(* Logix 5000 AddOnInstructionDefinition export Banner_LCA_Param_v4; software revision 33.00 *)

TYPE Banner_IOL_Port_v4 :   // UDT that has all of the data items necessary to communicate with a specific Port on a IO-Link Master
STRUCT
   Port_Controlled : INT;   // Each bit represents a port on an IO-Link Master. Set to 1 to tell AOI to control that port.
   Port_Activate : INT;   // Each bit represents a port on an IO-Link Master. When ON that port will process any commands in queue.
   Port_Read : INT;   // Each bit represents a port on an IO-Link Master. Used to determine when device AOI has requested a Read command.
   Port_Write : INT;   // Each bit represents a port on an IO-Link Master. Used to determine when device AOI has requested a Write command.
   Port_RW_Complete : INT;   // Each bit represents a port on an IO-Link Master. Tells device AOI that Read or Write request has been completed.
   Port_Device_Read : INT;
   Data_Transfer : SINT[190];   // Array to transfer data from IO-Master to device AOIs.
END_STRUCT
END_TYPE

TYPE Banner_LCA_Output_Settings_v4 :
STRUCT
   State : SINT;   // 0 = Normally Closed, 1 = Normally Open
   Off_Delay_Type : SINT;   // 0 = Leading Edge, 1 = Trailing Edge.
   Off_Delay : DINT;   // 0 to 65535 ms.
END_STRUCT
END_TYPE

TYPE Banner_LCA_RD_v4 :   // UDT with all of the Read only parameters for LCA.
STRUCT
   Master_Cycle_Time : INT;
   Min_Cycle_Time : INT;
   M_Sequence_Capability : INT;
   IO_Link_Version_ID : INT;
   Process_Data_Input_Length : INT;
   Process_Data_Output_Length : INT;
   Combined_Vendor_ID : DINT;   // IO-Link Vendor ID
   Vendor_ID1 : INT;
   Vendor_ID2 : INT;
   Combined_Device_ID : DINT;   // IO-Link Device ID
   Device_ID1 : INT;
   Device_ID2 : INT;
   Device_ID3 : INT;
   Serial_Number : STRING;
END_STRUCT
END_TYPE

TYPE Banner_LCA_Settings_v4 :
STRUCT
   Custom_Intensity : SINT;   // 0 to 100 %
   Custom_Flash_Rate : INT;   // Range 5 to 255 (.5 to 25.5 converted rate).
   Restrict_to_Gamut : SINT;   // 0 = Off, 1 = On.
END_STRUCT
END_TYPE

TYPE Banner_LCA_SP_Param_v4 :   // UDT for LCA with the Off State Parameters structure.
STRUCT
   Type : SINT;   // 0 = Off, 1 = Steady, 2 = Flash, 3 = Two Color Flash, 4 = Intensity Sweep, 5 = Color Sweep.
   Output : SINT;   // 0 = Off, 1 = On, 2 = Pattern.
   Pattern : SINT;   // 0 = Flash, 1 = Strobe, 2 = Three Pulse, 3 = SOS, 4 = Random.
   Speed : SINT;   // 0 = Slow, 1 = Medium, 2 = Fast, 3 = Custom.
   Off_Delay_Type : SINT;   // 0 = Leading Edge, 1 = Trailing Edge.
   Off_Delay : DINT;   // 0 to 65535 in ms. Length of time before the device returns to 'touch inactive' state after button is released.
   Color_1 : SINT;   // 0 = Green, 1 = Red, 2 = Orange, 3 = Amber, 4 = Yellow, 5 = Lime Green, 6 = Spring Green, 7 = Cyan, 8 = SKy Blue, 9 = Blue, 10 = Violet, 11 = Magenta, 12 = Rose, 13 = White, 14 Custom 1, 15 = Custom 2.
   Color_1_Intensity : SINT;   // 0 = High, 1 = Medium, 2 = Low, 3 = Off, 4 = Custom.
   Color_2 : SINT;   // 0 = Green, 1 = Red, 2 = Orange, 3 = Amber, 4 = Yellow, 5 = Lime Green, 6 = Spring Green, 7 = Cyan, 8 = SKy Blue, 9 = Blue, 10 = Violet, 11 = Magenta, 12 = Rose, 13 = White, 14 Custom 1, 15 = Custom 2.
   Color_2_Intensity : SINT;   // 0 = High, 1 = Medium, 2 = Low, 3 = Off, 4 = Custom.
END_STRUCT
END_TYPE

TYPE Banner_LCA_SP_v4 :
STRUCT
   Off : Banner_LCA_SP_Param_v4;
   On : Banner_LCA_SP_Param_v4;
   Hold : Banner_LCA_SP_Param_v4;
END_STRUCT
END_TYPE

TYPE Banner_LCA_Touch_Settings_v4 :
STRUCT
   Touch_Sensitivity : SINT;   // 0 = Low, 1 = High.
   Function : SINT[6];   // 0 = Momentary, 1 = Latched.
   Hold : SINT[6];   // 0 = Disabled, 1 = Enabled.
END_STRUCT
END_TYPE

TYPE Banner_LCA_v4 :   // UDT with all of the parameters for LCA.
STRUCT
   Initial_Global_Read : BOOL;   // Determines if all of the IO-Link data has been read into the PLC yet
   Command : INT;   // Value placed in here will activate a read or write to a specifc IO-Link Index
   Read : Banner_LCA_RD_v4;   // All read data
   Write : Banner_LCA_WD_v4;   // All data that can be written to.
   Archive : Banner_LCA_WD_v4;   // Archive of the write data.
   Reset : BOOL;
END_STRUCT
END_TYPE

TYPE Banner_LCA_WD_v4 :   // UDT that stores the Write Data for a LCA.
STRUCT
   System_Command : INT;   // See IODD file for list of commands that can be activated via the System Command interface
   Parameter_Access_Lock : SINT;   // Write access to all read/write parameters is block when this bit is ON.
   Data_Storage_Lock : SINT;   // Data storage mechanism is inhibited when bit is ON.
   Local_Parameterization_Lock : SINT;   // Parameteriation via local control elementes is inhibited.
   Local_User_Interface_Lock : SINT;   // Operation of the hmi on the device is disabled.
   Operation_Mode : SINT;   // 0 = Multicolor, 1 = Four State Full Logic, 2 = Advanced, 3 = LED Control, 4 = Demo.
   Animation_Settings : Banner_LCA_Settings_v4;
   Touch_Settings : Banner_LCA_Touch_Settings_v4;
   Output_Settings : Banner_LCA_Output_Settings_v4;
   State_Parameters : Banner_LCA_SP_v4[6];   // State Parameters. 1 through 5 will have values.
   CC1_Red : INT;   // 0-255. Custom 1 Red.
   CC1_Green : INT;   // 0-255. Custom 1 Green.
   CC1_Blue : INT;   // 0-255. Custom 1 Blue.
   CC2_Red : INT;   // 0-255. Custom 2 Red.
   CC2_Green : INT;   // 0-255. Custom 2 Green.
   CC_Blue : INT;   // 0-255. Custom 2 Blue.
END_STRUCT
END_TYPE

ADD_ON_INSTRUCTION Banner_LCA_Param_SP_In_v4   (* revision 4.0 *)
VAR_INPUT
   Byte1 : SINT; {required}
   Byte2 : SINT; {required}
   Byte3 : SINT; {required}
   Byte4 : SINT; {required}
   Byte5 : SINT; {required}
   Byte6 : SINT; {required}
END_VAR
VAR_IN_OUT
   Data : Banner_LCA_SP_Param_v4; {required}
END_VAR

ROUTINE Logic   (* ladder *)
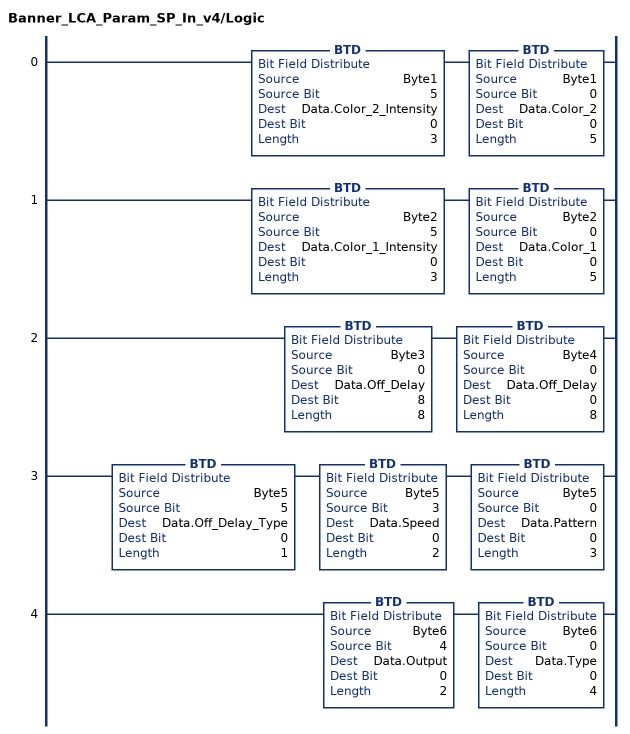
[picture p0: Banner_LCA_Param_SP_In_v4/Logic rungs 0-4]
   0: BTD(Byte1,5,Data.Color_2_Intensity,0,3)BTD(Byte1,0,Data.Color_2,0,5);
   1: BTD(Byte2,5,Data.Color_1_Intensity,0,3)BTD(Byte2,0,Data.Color_1,0,5);
   2: BTD(Byte3,0,Data.Off_Delay,8,8)BTD(Byte4,0,Data.Off_Delay,0,8);
   3: BTD(Byte5,5,Data.Off_Delay_Type,0,1)BTD(Byte5,3,Data.Speed,0,2)BTD(Byte5,0,Data.Pattern,0,3);
   4: BTD(Byte6,4,Data.Output,0,2)BTD(Byte6,0,Data.Type,0,4);
END_ROUTINE
END_ADD_ON_INSTRUCTION

ADD_ON_INSTRUCTION Banner_LCA_Param_SP_Out_v4   (* revision 4.0 *)
VAR_OUTPUT
   Byte1 : SINT; {required}
   Byte2 : SINT; {required}
   Byte3 : SINT; {required}
   Byte4 : SINT; {required}
   Byte5 : SINT; {required}
   Byte6 : SINT; {required}
END_VAR
VAR_IN_OUT
   Data : Banner_LCA_SP_Param_v4; {required}
END_VAR

ROUTINE Logic   (* ladder *)
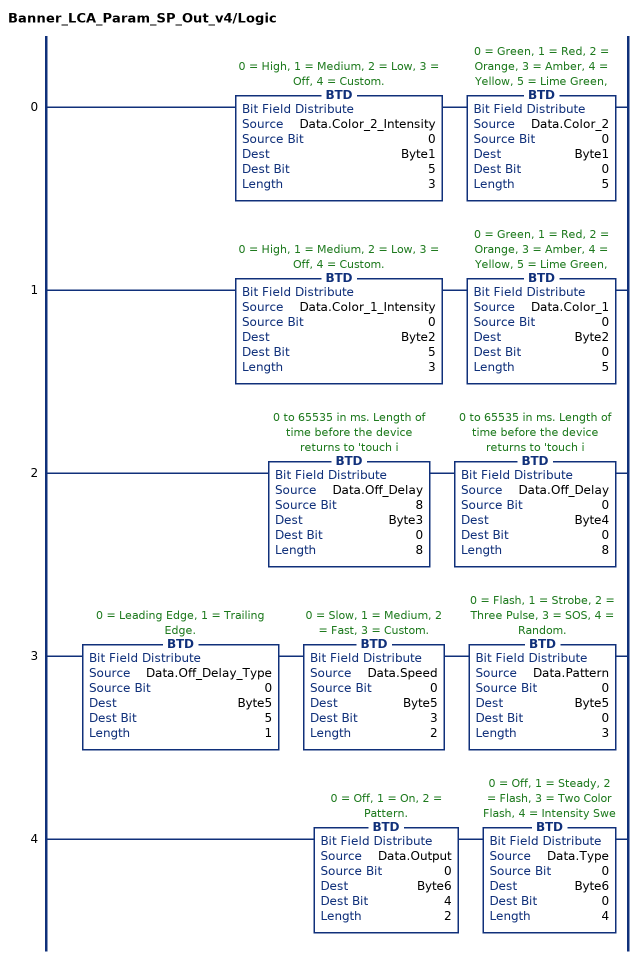
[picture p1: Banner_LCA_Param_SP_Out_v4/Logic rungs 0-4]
   0: BTD(Data.Color_2_Intensity,0,Byte1,5,3)BTD(Data.Color_2,0,Byte1,0,5);
   1: BTD(Data.Color_1_Intensity,0,Byte2,5,3)BTD(Data.Color_1,0,Byte2,0,5);
   2: BTD(Data.Off_Delay,8,Byte3,0,8)BTD(Data.Off_Delay,0,Byte4,0,8);
   3: BTD(Data.Off_Delay_Type,0,Byte5,5,1)BTD(Data.Speed,0,Byte5,3,2)BTD(Data.Pattern,0,Byte5,0,3);
   4: BTD(Data.Output,0,Byte6,4,2)BTD(Data.Type,0,Byte6,0,4);
END_ROUTINE
END_ADD_ON_INSTRUCTION

ADD_ON_INSTRUCTION Banner_LCA_Param_v4   (* revision 4.0, vendor Banner Engineering *)
// AOI to read and write parameter data to an IO-Link LCA.
VAR_IN_OUT
   LCA : Banner_LCA_v4; {required}
   Port_Data : Banner_IOL_Port_v4; {required}
END_VAR
VAR_INPUT
   Port : DINT; {required}
END_VAR
VAR
   Local_Control : DINT; {access None}
   Global_Read_Command_Value : INT; {access None}
   Global_Write_Command_Value : INT; {access None}
   Command_Being_Processed : BOOL; {access None}
   Update_Archive : BOOL; {access None}
   Index_Write_Control : DINT; {access None}
   Index_Write_Inprocess : INT; {access None}
   Temp_Excess_Gain : DINT[2]; {access None}
   Inprocess_Index : DINT; {access None}
   SP_Index : DINT; {access None}   // State Parameters Index
   SP_Write_Index : DINT; {access None}
   SP_R_Index : DINT; {access None}
   SP_W_Index : DINT; {access None}
   StatusIn : Banner_LCA_Param_SP_In_v4[3]; {access None}
   OffArchive : DINT; {access None}
   OffData : DINT; {access None}
   HoldData : DINT; {access None}
   HoldArchive : DINT; {access None}
   OnData : DINT; {access None}
   OnArchive : DINT; {access None}
   StatusOut : Banner_LCA_Param_SP_Out_v4[3]; {access None}
   W_SP_Index : DINT; {access None}
END_VAR

ROUTINE Logic   (* ladder *)
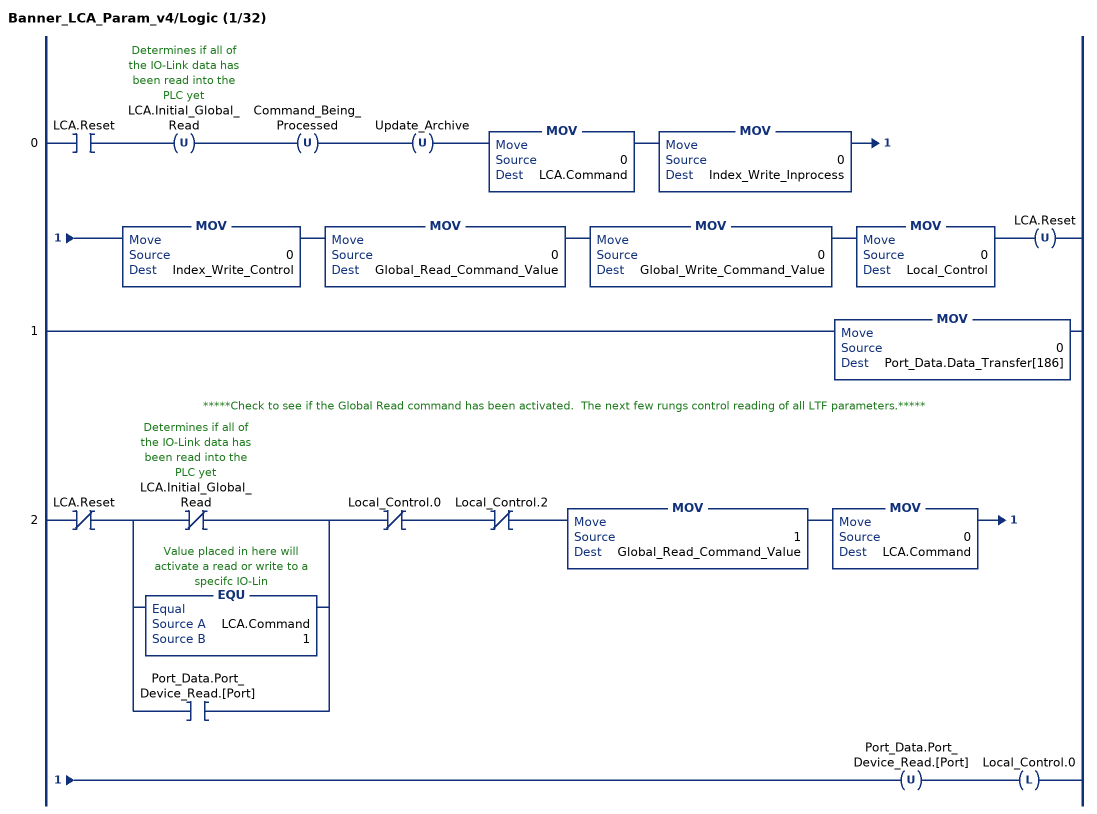
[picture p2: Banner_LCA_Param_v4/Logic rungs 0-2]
   0: XIC(LCA.Reset)OTU(LCA.Initial_Global_Read)OTU(Command_Being_Processed)OTU(Update_Archive)MOV(0,LCA.Command)MOV(0,Index_Write_Inprocess)MOV(0,Index_Write_Control)MOV(0,Global_Read_Command_Value)MOV(0,Global_Write_Command_Value)MOV(0,Local_Control)OTU(LCA.Reset);
   1: MOV(0,Port_Data.Data_Transfer[186]);
   // *****Check to see if the Global Read command has been activated.  The next few rungs control reading of all LTF parameters.*****
   2: XIO(LCA.Reset)[XIO(LCA.Initial_Global_Read) ,EQU(LCA.Command,1) ,XIC(Port_Data.Port_Device_Read.[Port]) ]XIO(Local_Control.0)XIO(Local_Control.2)MOV(1,Global_Read_Command_Value)MOV(0,LCA.Command)OTU(Port_Data.Port_Device_Read.[Port])OTL(Local_Control.0);
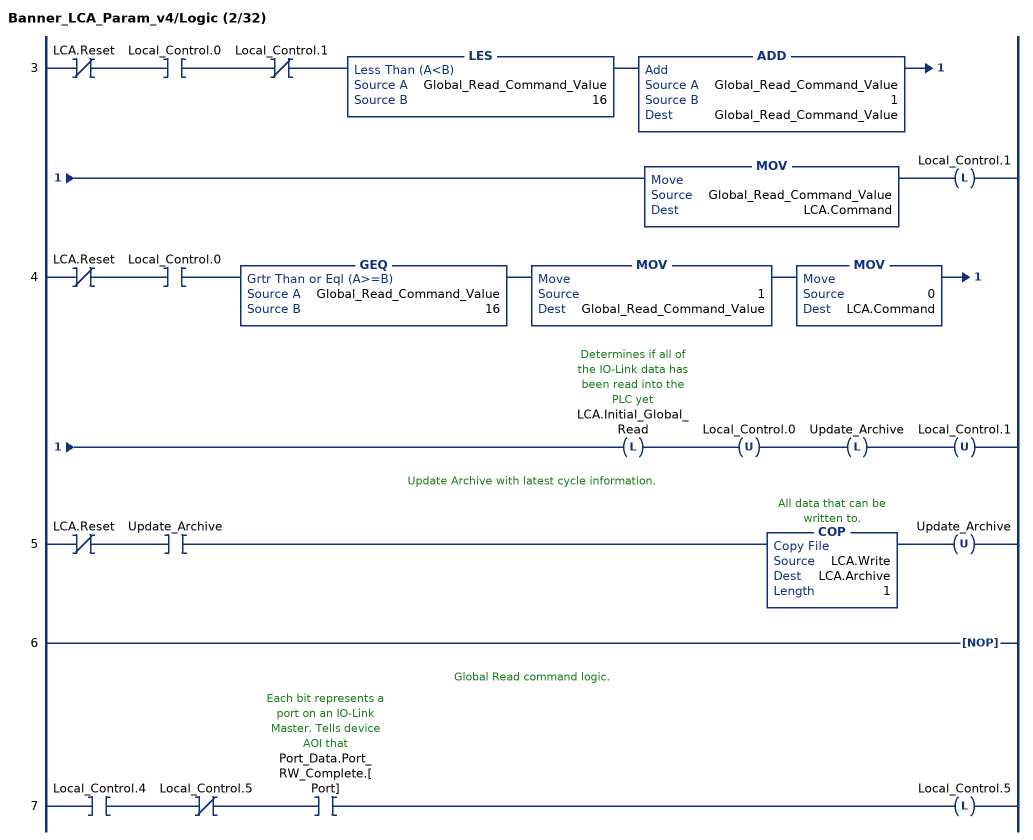
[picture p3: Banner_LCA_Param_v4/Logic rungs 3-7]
   3: XIO(LCA.Reset)XIC(Local_Control.0)XIO(Local_Control.1)LES(Global_Read_Command_Value,16)ADD(Global_Read_Command_Value,1,Global_Read_Command_Value)MOV(Global_Read_Command_Value,LCA.Command)OTL(Local_Control.1);
   4: XIO(LCA.Reset)XIC(Local_Control.0)GEQ(Global_Read_Command_Value,16)MOV(1,Global_Read_Command_Value)MOV(0,LCA.Command)OTL(LCA.Initial_Global_Read)OTU(Local_Control.0)OTL(Update_Archive)OTU(Local_Control.1);
   // Update Archive with latest cycle information.
   5: XIO(LCA.Reset)XIC(Update_Archive)COP(LCA.Write,LCA.Archive,1)OTU(Update_Archive);
   6: NOP();
   // Global Read command logic.
   7: XIC(Local_Control.4)XIO(Local_Control.5)XIC(Port_Data.Port_RW_Complete.[Port])OTL(Local_Control.5);
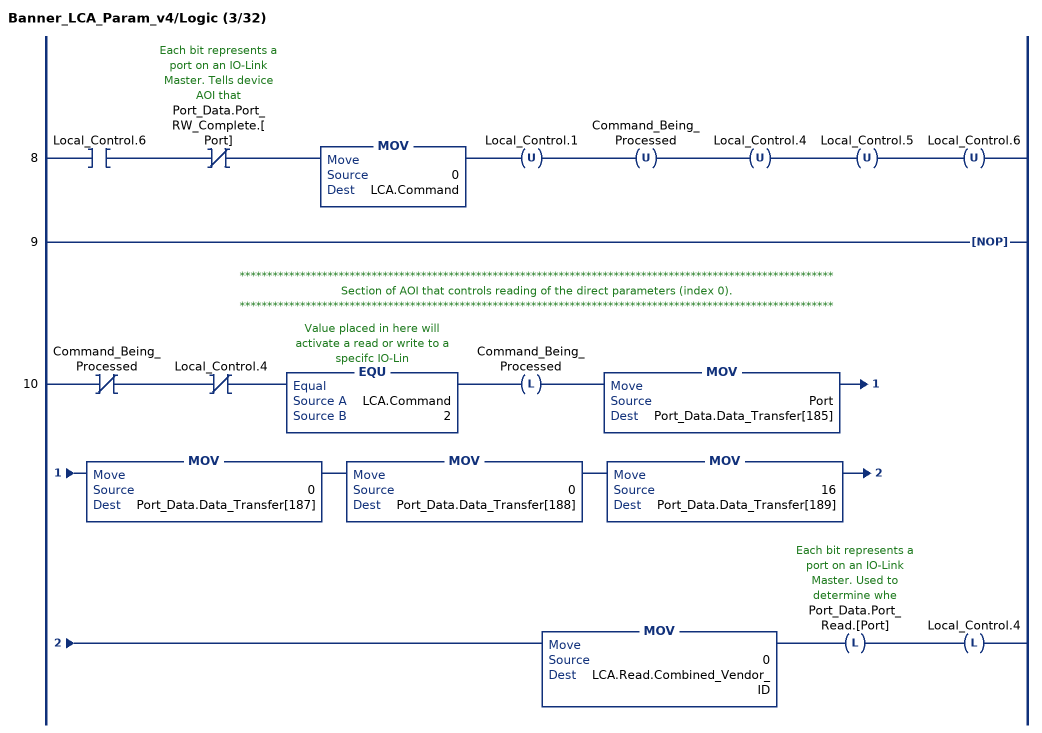
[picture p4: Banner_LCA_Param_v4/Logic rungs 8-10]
   8: XIC(Local_Control.6)XIO(Port_Data.Port_RW_Complete.[Port])MOV(0,LCA.Command)OTU(Local_Control.1)OTU(Command_Being_Processed)OTU(Local_Control.4)OTU(Local_Control.5)OTU(Local_Control.6);
   9: NOP();
   // ************************************************************************************************************
   // Section of AOI that controls reading of the direct parameters (index 0).
   // ************************************************************************************************************
   10: XIO(Command_Being_Processed)XIO(Local_Control.4)EQU(LCA.Command,2)OTL(Command_Being_Processed)MOV(Port,Port_Data.Data_Transfer[185])MOV(0,Port_Data.Data_Transfer[187])MOV(0,Port_Data.Data_Transfer[188])MOV(16,Port_Data.Data_Transfer[189])MOV(0,LCA.Read.Combined_Vendor_ID)OTL(Port_Data.Port_Read.[Port])OTL(Local_Control.4);
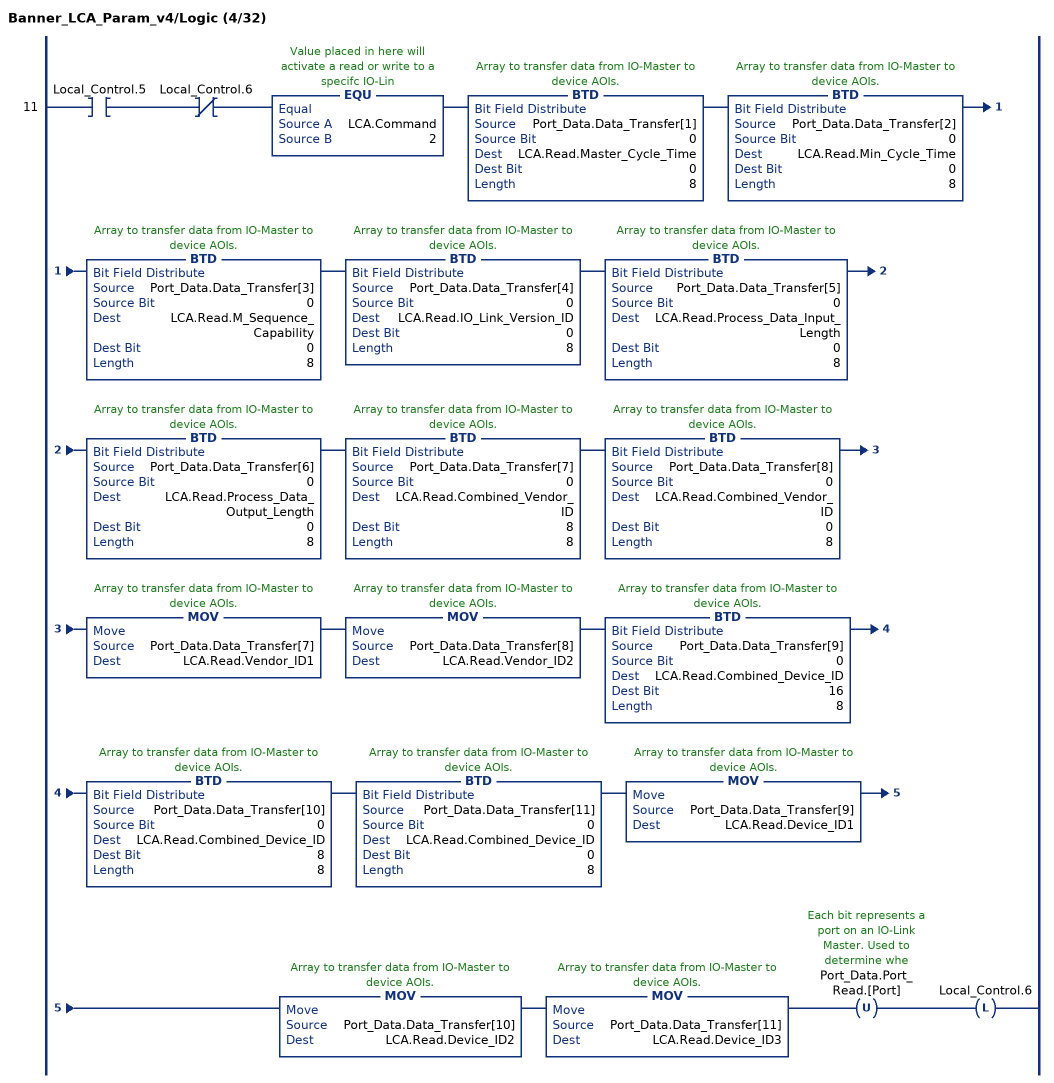
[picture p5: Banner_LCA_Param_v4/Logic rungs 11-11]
   11: XIC(Local_Control.5)XIO(Local_Control.6)EQU(LCA.Command,2)BTD(Port_Data.Data_Transfer[1],0,LCA.Read.Master_Cycle_Time,0,8)BTD(Port_Data.Data_Transfer[2],0,LCA.Read.Min_Cycle_Time,0,8)BTD(Port_Data.Data_Transfer[3],0,LCA.Read.M_Sequence_Capability,0,8)BTD(Port_Data.Data_Transfer[4],0,LCA.Read.IO_Link_Version_ID,0,8)BTD(Port_Data.Data_Transfer[5],0,LCA.Read.Process_Data_Input_Length,0,8)BTD(Port_Data.Data_Transfer[6],0,LCA.Read.Process_Data_Output_Length,0,8)BTD(Port_Data.Data_Transfer[7],0,LCA.Read.Combined_Vendor_ID,8,8)BTD(Port_Data.Data_Transfer[8],0,LCA.Read.Combined_Vendor_ID,0,8)MOV(Port_Data.Data_Transfer[7],LCA.Read.Vendor_ID1)MOV(Port_Data.Data_Transfer[8],LCA.Read.Vendor_ID2)BTD(Port_Data.Data_Transfer[9],0,LCA.Read.Combined_Device_ID,16,8)BTD(Port_Data.Data_Transfer[10],0,LCA.Read.Combined_Device_ID,8,8)BTD(Port_Data.Data_Transfer[11],0,LCA.Read.Combined_Device_ID,0,8)MOV(Port_Data.Data_Transfer[9],LCA.Read.Device_ID1)MOV(Port_Data.Data_Transfer[10],LCA.Read.Device_ID2)MOV(Port_Data.Data_Transfer[11],LCA.Read.Device_ID3)OTU(Port_Data.Port_Read.[Port])OTL(Local_Control.6);
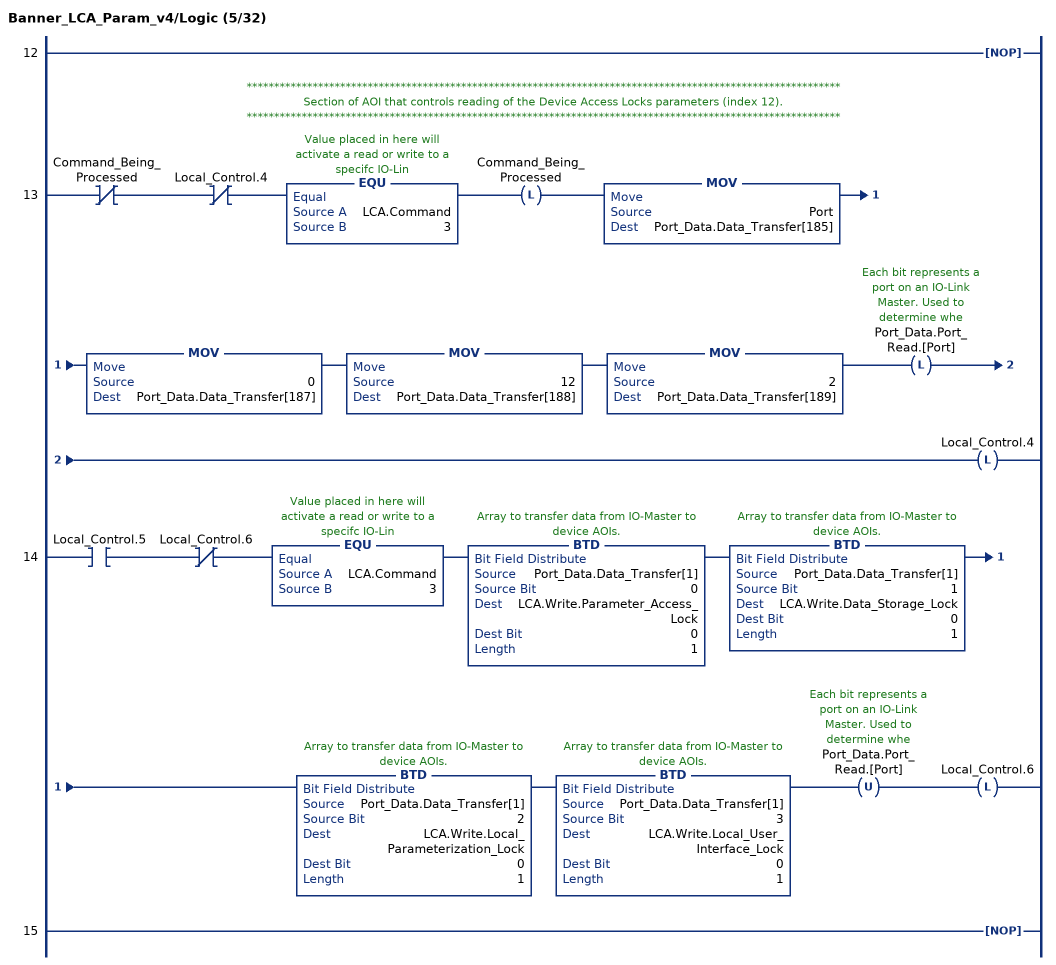
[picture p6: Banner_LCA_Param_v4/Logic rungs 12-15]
   12: NOP();
   // ************************************************************************************************************
   // Section of AOI that controls reading of the Device Access Locks parameters (index 12).
   // ************************************************************************************************************
   13: XIO(Command_Being_Processed)XIO(Local_Control.4)EQU(LCA.Command,3)OTL(Command_Being_Processed)MOV(Port,Port_Data.Data_Transfer[185])MOV(0,Port_Data.Data_Transfer[187])MOV(12,Port_Data.Data_Transfer[188])MOV(2,Port_Data.Data_Transfer[189])OTL(Port_Data.Port_Read.[Port])OTL(Local_Control.4);
   14: XIC(Local_Control.5)XIO(Local_Control.6)EQU(LCA.Command,3)BTD(Port_Data.Data_Transfer[1],0,LCA.Write.Parameter_Access_Lock,0,1)BTD(Port_Data.Data_Transfer[1],1,LCA.Write.Data_Storage_Lock,0,1)BTD(Port_Data.Data_Transfer[1],2,LCA.Write.Local_Parameterization_Lock,0,1)BTD(Port_Data.Data_Transfer[1],3,LCA.Write.Local_User_Interface_Lock,0,1)OTU(Port_Data.Port_Read.[Port])OTL(Local_Control.6);
   15: NOP();
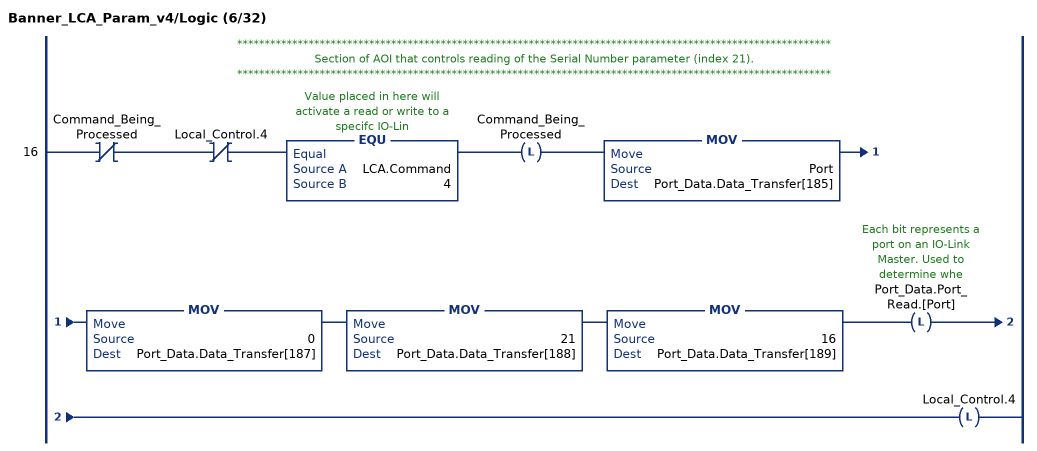
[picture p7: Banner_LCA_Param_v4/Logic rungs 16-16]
   // ************************************************************************************************************
   // Section of AOI that controls reading of the Serial Number parameter (index 21).
   // ************************************************************************************************************
   16: XIO(Command_Being_Processed)XIO(Local_Control.4)EQU(LCA.Command,4)OTL(Command_Being_Processed)MOV(Port,Port_Data.Data_Transfer[185])MOV(0,Port_Data.Data_Transfer[187])MOV(21,Port_Data.Data_Transfer[188])MOV(16,Port_Data.Data_Transfer[189])OTL(Port_Data.Port_Read.[Port])OTL(Local_Control.4);
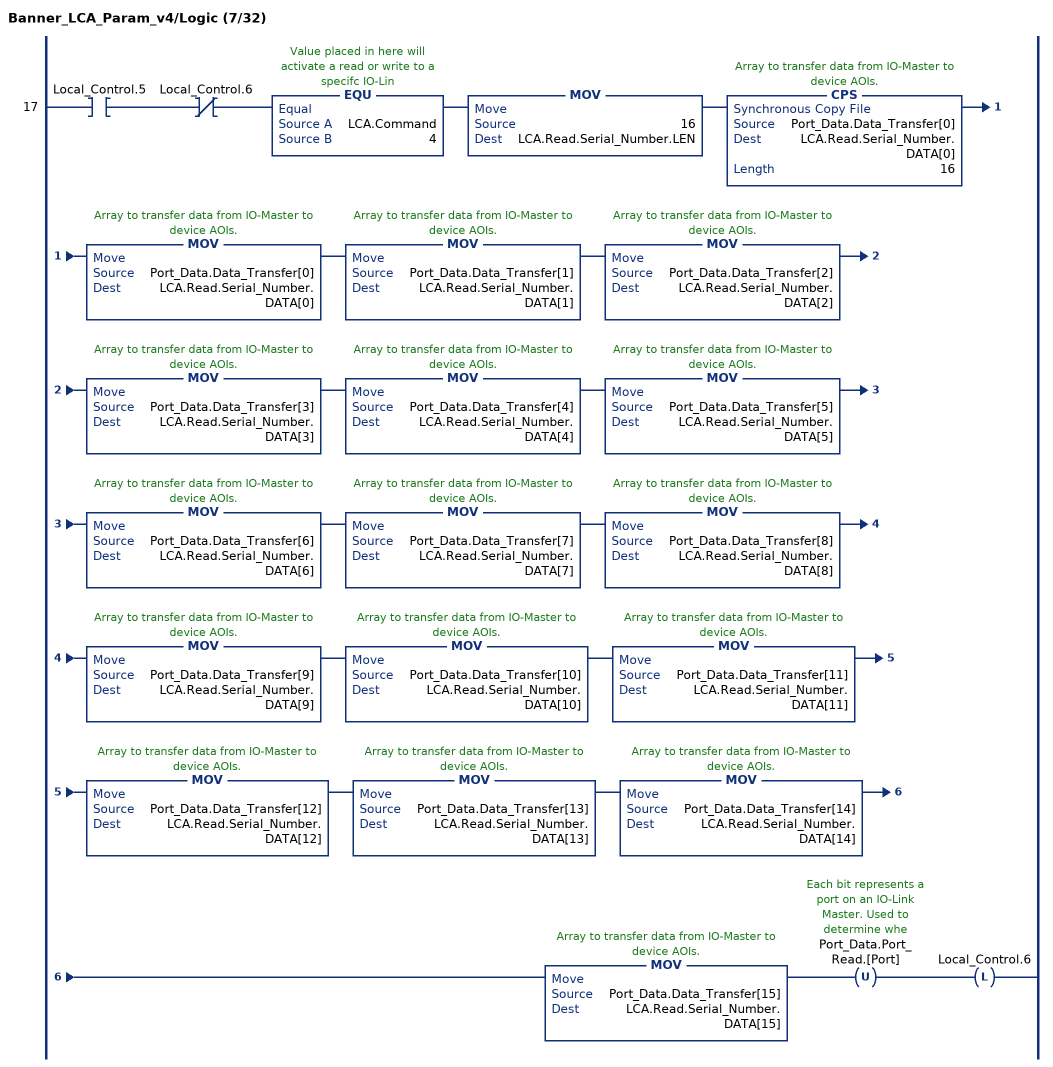
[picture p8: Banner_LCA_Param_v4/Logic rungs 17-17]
   17: XIC(Local_Control.5)XIO(Local_Control.6)EQU(LCA.Command,4)MOV(16,LCA.Read.Serial_Number.LEN)CPS(Port_Data.Data_Transfer[0],LCA.Read.Serial_Number.DATA[0],16)MOV(Port_Data.Data_Transfer[0],LCA.Read.Serial_Number.DATA[0])MOV(Port_Data.Data_Transfer[1],LCA.Read.Serial_Number.DATA[1])MOV(Port_Data.Data_Transfer[2],LCA.Read.Serial_Number.DATA[2])MOV(Port_Data.Data_Transfer[3],LCA.Read.Serial_Number.DATA[3])MOV(Port_Data.Data_Transfer[4],LCA.Read.Serial_Number.DATA[4])MOV(Port_Data.Data_Transfer[5],LCA.Read.Serial_Number.DATA[5])MOV(Port_Data.Data_Transfer[6],LCA.Read.Serial_Number.DATA[6])MOV(Port_Data.Data_Transfer[7],LCA.Read.Serial_Number.DATA[7])MOV(Port_Data.Data_Transfer[8],LCA.Read.Serial_Number.DATA[8])MOV(Port_Data.Data_Transfer[9],LCA.Read.Serial_Number.DATA[9])MOV(Port_Data.Data_Transfer[10],LCA.Read.Serial_Number.DATA[10])MOV(Port_Data.Data_Transfer[11],LCA.Read.Serial_Number.DATA[11])MOV(Port_Data.Data_Transfer[12],LCA.Read.Serial_Number.DATA[12])MOV(Port_Data.Data_Transfer[13],LCA.Read.Serial_Number.DATA[13])MOV(Port_Data.Data_Transfer[14],LCA.Read.Serial_Number.DATA[14])MOV(Port_Data.Data_Transfer[15],LCA.Read.Serial_Number.DATA[15])OTU(Port_Data.Port_Read.[Port])OTL(Local_Control.6);
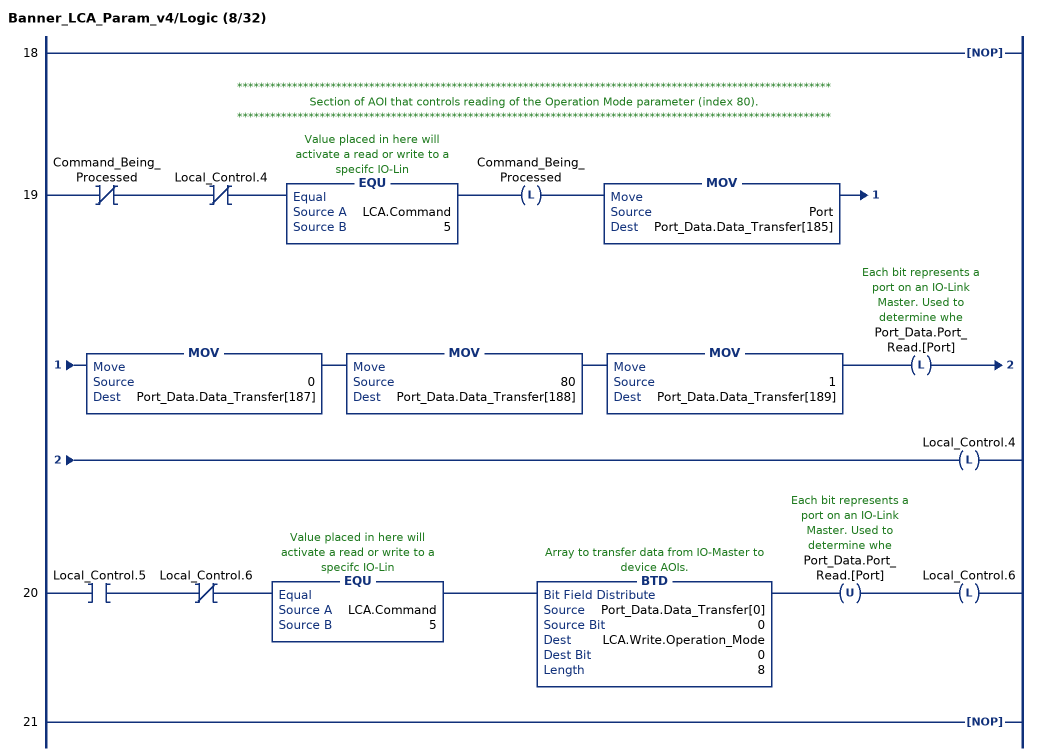
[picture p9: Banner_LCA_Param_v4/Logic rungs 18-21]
   18: NOP();
   // ************************************************************************************************************
   // Section of AOI that controls reading of the Operation Mode parameter (index 80).
   // ************************************************************************************************************
   19: XIO(Command_Being_Processed)XIO(Local_Control.4)EQU(LCA.Command,5)OTL(Command_Being_Processed)MOV(Port,Port_Data.Data_Transfer[185])MOV(0,Port_Data.Data_Transfer[187])MOV(80,Port_Data.Data_Transfer[188])MOV(1,Port_Data.Data_Transfer[189])OTL(Port_Data.Port_Read.[Port])OTL(Local_Control.4);
   20: XIC(Local_Control.5)XIO(Local_Control.6)EQU(LCA.Command,5)BTD(Port_Data.Data_Transfer[0],0,LCA.Write.Operation_Mode,0,8)OTU(Port_Data.Port_Read.[Port])OTL(Local_Control.6);
   21: NOP();
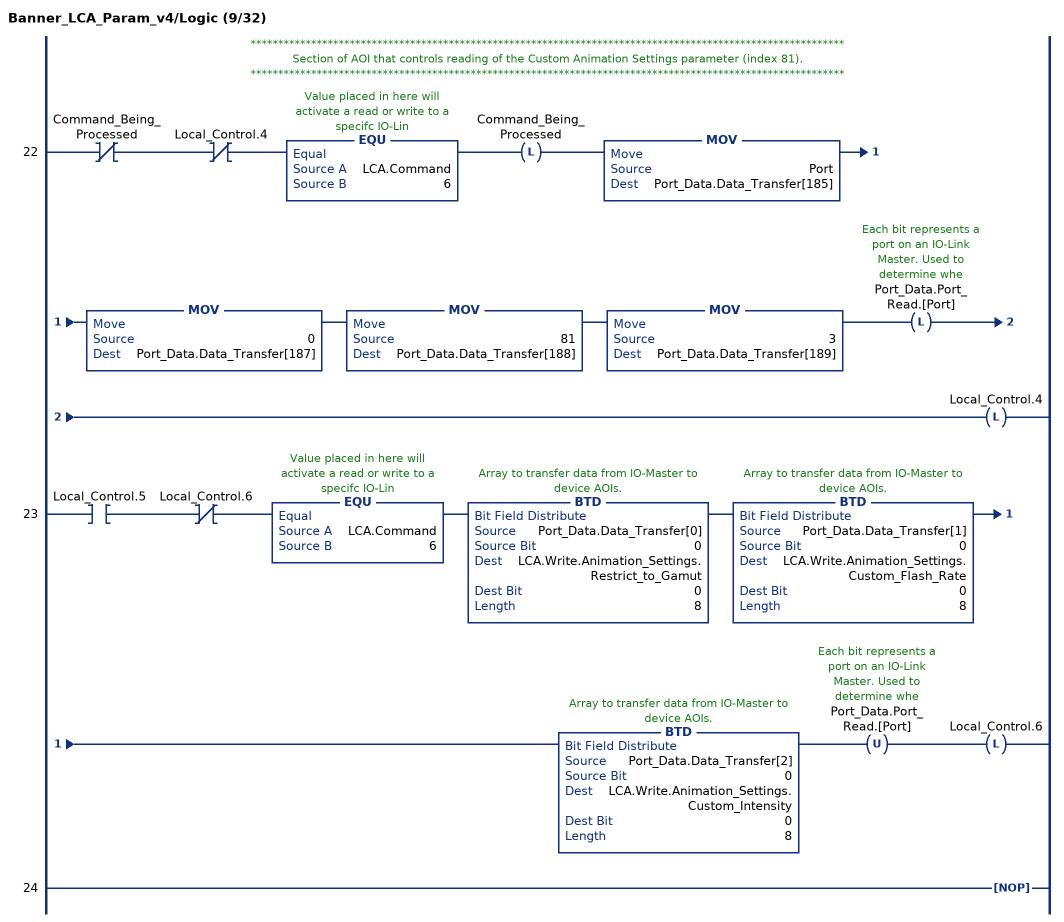
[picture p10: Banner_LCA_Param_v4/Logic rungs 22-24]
   // ************************************************************************************************************
   // Section of AOI that controls reading of the Custom Animation Settings parameter (index 81).
   // ************************************************************************************************************
   22: XIO(Command_Being_Processed)XIO(Local_Control.4)EQU(LCA.Command,6)OTL(Command_Being_Processed)MOV(Port,Port_Data.Data_Transfer[185])MOV(0,Port_Data.Data_Transfer[187])MOV(81,Port_Data.Data_Transfer[188])MOV(3,Port_Data.Data_Transfer[189])OTL(Port_Data.Port_Read.[Port])OTL(Local_Control.4);
   23: XIC(Local_Control.5)XIO(Local_Control.6)EQU(LCA.Command,6)BTD(Port_Data.Data_Transfer[0],0,LCA.Write.Animation_Settings.Restrict_to_Gamut,0,8)BTD(Port_Data.Data_Transfer[1],0,LCA.Write.Animation_Settings.Custom_Flash_Rate,0,8)BTD(Port_Data.Data_Transfer[2],0,LCA.Write.Animation_Settings.Custom_Intensity,0,8)OTU(Port_Data.Port_Read.[Port])OTL(Local_Control.6);
   24: NOP();
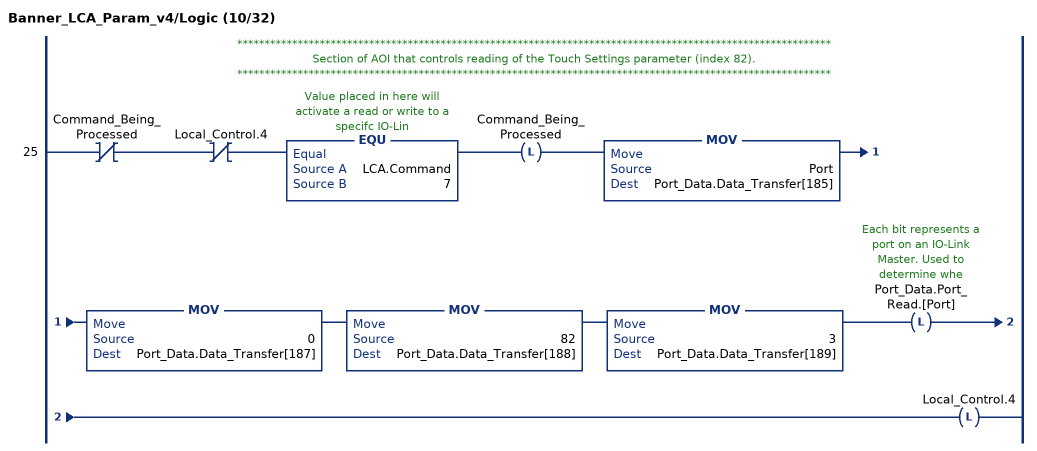
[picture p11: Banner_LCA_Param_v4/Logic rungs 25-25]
   // ************************************************************************************************************
   // Section of AOI that controls reading of the Touch Settings parameter (index 82).
   // ************************************************************************************************************
   25: XIO(Command_Being_Processed)XIO(Local_Control.4)EQU(LCA.Command,7)OTL(Command_Being_Processed)MOV(Port,Port_Data.Data_Transfer[185])MOV(0,Port_Data.Data_Transfer[187])MOV(82,Port_Data.Data_Transfer[188])MOV(3,Port_Data.Data_Transfer[189])OTL(Port_Data.Port_Read.[Port])OTL(Local_Control.4);
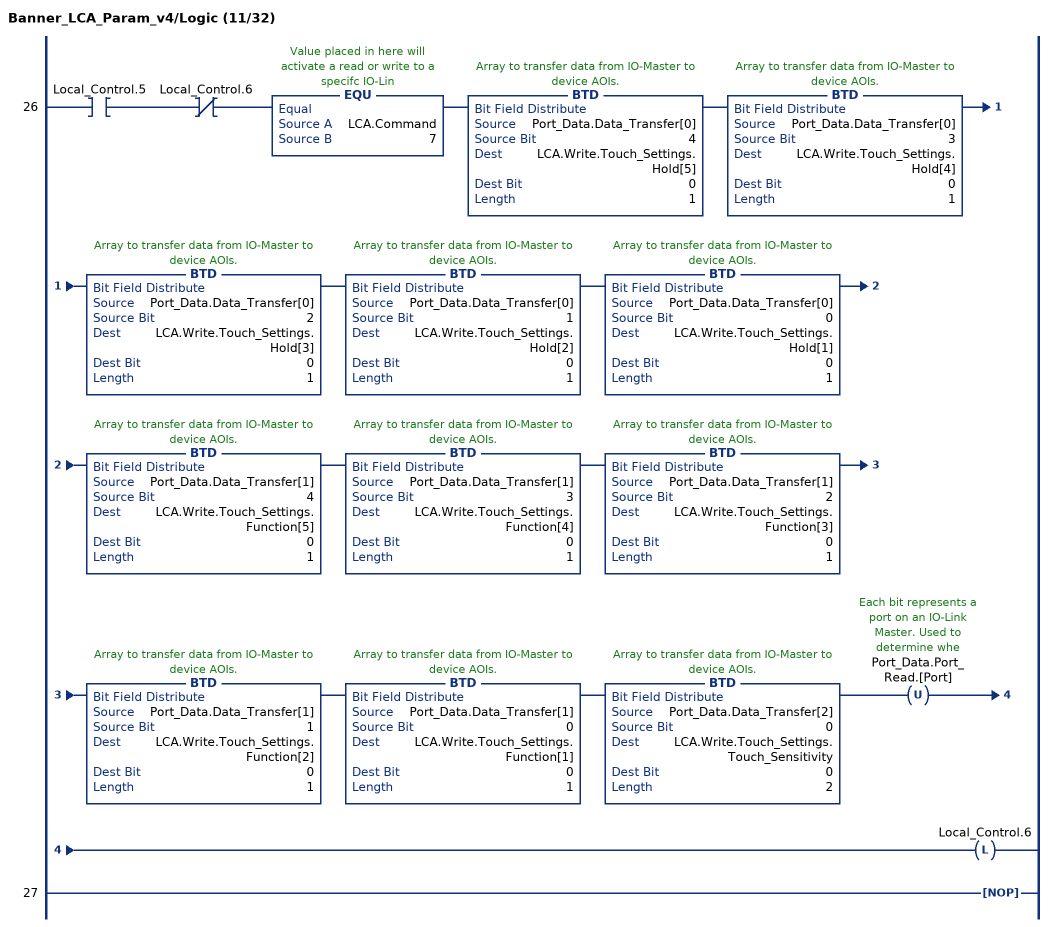
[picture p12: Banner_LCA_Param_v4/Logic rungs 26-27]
   26: XIC(Local_Control.5)XIO(Local_Control.6)EQU(LCA.Command,7)BTD(Port_Data.Data_Transfer[0],4,LCA.Write.Touch_Settings.Hold[5],0,1)BTD(Port_Data.Data_Transfer[0],3,LCA.Write.Touch_Settings.Hold[4],0,1)BTD(Port_Data.Data_Transfer[0],2,LCA.Write.Touch_Settings.Hold[3],0,1)BTD(Port_Data.Data_Transfer[0],1,LCA.Write.Touch_Settings.Hold[2],0,1)BTD(Port_Data.Data_Transfer[0],0,LCA.Write.Touch_Settings.Hold[1],0,1)BTD(Port_Data.Data_Transfer[1],4,LCA.Write.Touch_Settings.Function[5],0,1)BTD(Port_Data.Data_Transfer[1],3,LCA.Write.Touch_Settings.Function[4],0,1)BTD(Port_Data.Data_Transfer[1],2,LCA.Write.Touch_Settings.Function[3],0,1)BTD(Port_Data.Data_Transfer[1],1,LCA.Write.Touch_Settings.Function[2],0,1)BTD(Port_Data.Data_Transfer[1],0,LCA.Write.Touch_Settings.Function[1],0,1)BTD(Port_Data.Data_Transfer[2],0,LCA.Write.Touch_Settings.Touch_Sensitivity,0,2)OTU(Port_Data.Port_Read.[Port])OTL(Local_Control.6);
   27: NOP();
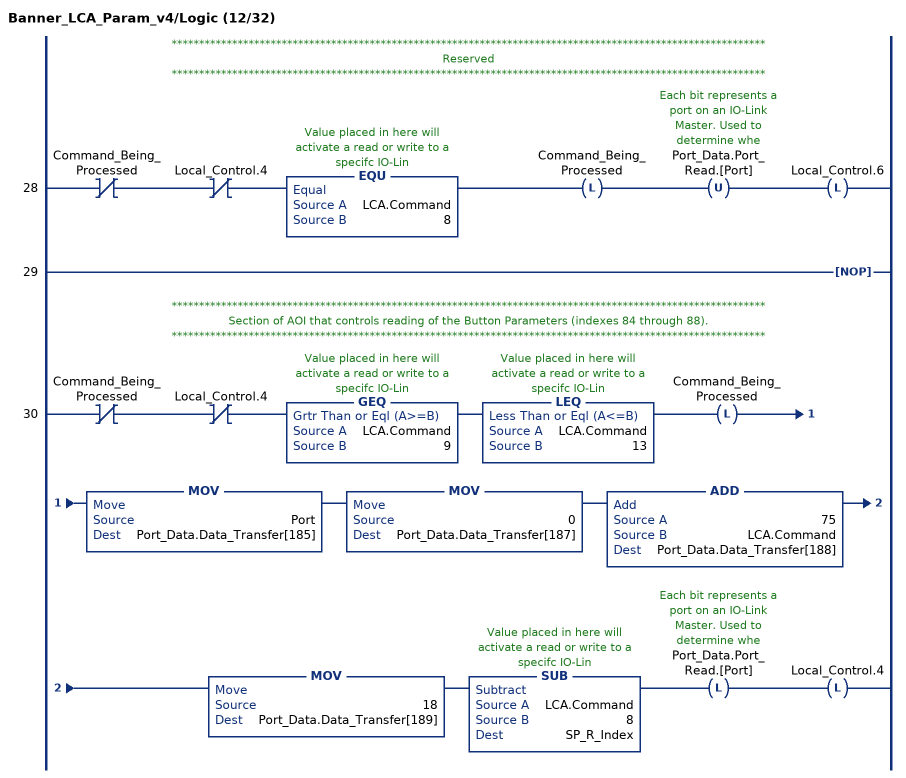
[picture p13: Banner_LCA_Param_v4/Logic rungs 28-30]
   // ************************************************************************************************************
   // Reserved
   // ************************************************************************************************************
   28: XIO(Command_Being_Processed)XIO(Local_Control.4)EQU(LCA.Command,8)OTL(Command_Being_Processed)OTU(Port_Data.Port_Read.[Port])OTL(Local_Control.6);
   29: NOP();
   // ************************************************************************************************************
   // Section of AOI that controls reading of the Button Parameters (indexes 84 through 88).
   // ************************************************************************************************************
   30: XIO(Command_Being_Processed)XIO(Local_Control.4)GEQ(LCA.Command,9)LEQ(LCA.Command,13)OTL(Command_Being_Processed)MOV(Port,Port_Data.Data_Transfer[185])MOV(0,Port_Data.Data_Transfer[187])ADD(75,LCA.Command,Port_Data.Data_Transfer[188])MOV(18,Port_Data.Data_Transfer[189])SUB(LCA.Command,8,SP_R_Index)OTL(Port_Data.Port_Read.[Port])OTL(Local_Control.4);
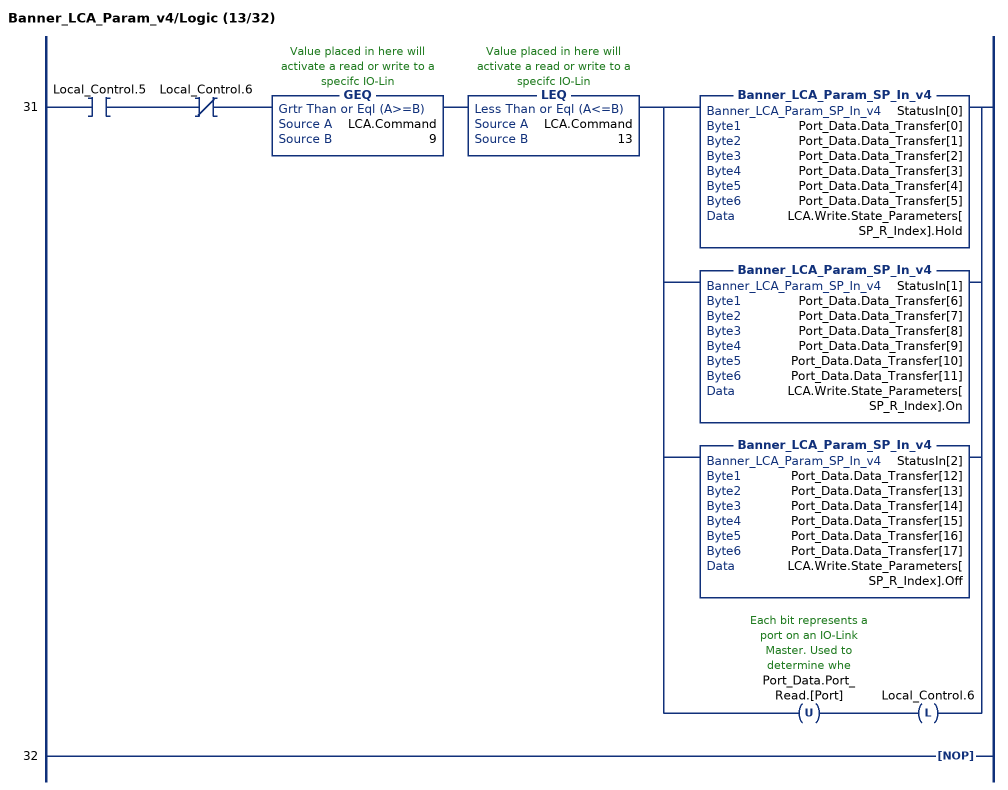
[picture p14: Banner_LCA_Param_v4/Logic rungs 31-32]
   31: XIC(Local_Control.5)XIO(Local_Control.6)GEQ(LCA.Command,9)LEQ(LCA.Command,13)[Banner_LCA_Param_SP_In_v4(StatusIn[0],Port_Data.Data_Transfer[0],Port_Data.Data_Transfer[1],Port_Data.Data_Transfer[2],Port_Data.Data_Transfer[3],Port_Data.Data_Transfer[4],Port_Data.Data_Transfer[5],LCA.Write.State_Parameters[SP_R_Index].Hold) ,Banner_LCA_Param_SP_In_v4(StatusIn[1],Port_Data.Data_Transfer[6],Port_Data.Data_Transfer[7],Port_Data.Data_Transfer[8],Port_Data.Data_Transfer[9],Port_Data.Data_Transfer[10],Port_Data.Data_Transfer[11],LCA.Write.State_Parameters[SP_R_Index].On) ,Banner_LCA_Param_SP_In_v4(StatusIn[2],Port_Data.Data_Transfer[12],Port_Data.Data_Transfer[13],Port_Data.Data_Transfer[14],Port_Data.Data_Transfer[15],Port_Data.Data_Transfer[16],Port_Data.Data_Transfer[17],LCA.Write.State_Parameters[SP_R_Index].Off) ,OTU(Port_Data.Port_Read.[Port]) OTL(Local_Control.6) ];
   32: NOP();
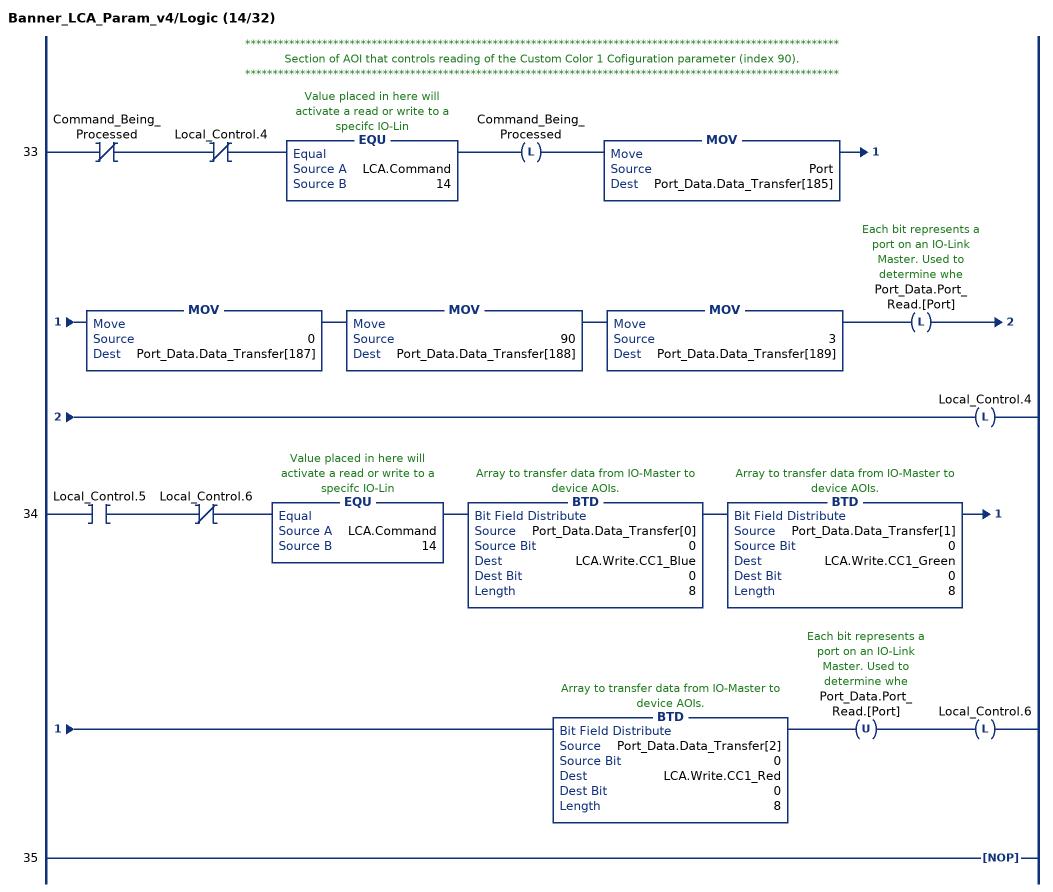
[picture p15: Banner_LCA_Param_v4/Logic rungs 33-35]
   // ************************************************************************************************************
   // Section of AOI that controls reading of the Custom Color 1 Cofiguration parameter (index 90).
   // ************************************************************************************************************
   33: XIO(Command_Being_Processed)XIO(Local_Control.4)EQU(LCA.Command,14)OTL(Command_Being_Processed)MOV(Port,Port_Data.Data_Transfer[185])MOV(0,Port_Data.Data_Transfer[187])MOV(90,Port_Data.Data_Transfer[188])MOV(3,Port_Data.Data_Transfer[189])OTL(Port_Data.Port_Read.[Port])OTL(Local_Control.4);
   34: XIC(Local_Control.5)XIO(Local_Control.6)EQU(LCA.Command,14)BTD(Port_Data.Data_Transfer[0],0,LCA.Write.CC1_Blue,0,8)BTD(Port_Data.Data_Transfer[1],0,LCA.Write.CC1_Green,0,8)BTD(Port_Data.Data_Transfer[2],0,LCA.Write.CC1_Red,0,8)OTU(Port_Data.Port_Read.[Port])OTL(Local_Control.6);
   35: NOP();
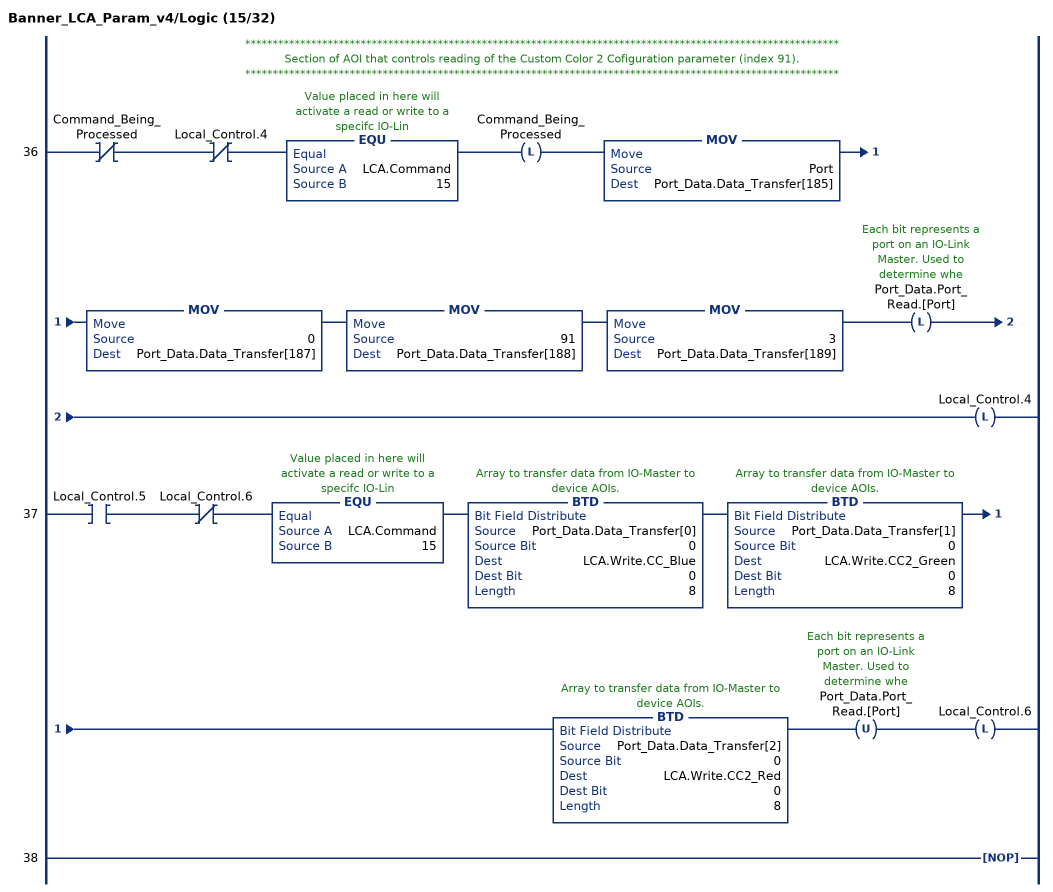
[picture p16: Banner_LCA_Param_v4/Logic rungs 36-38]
   // ************************************************************************************************************
   // Section of AOI that controls reading of the Custom Color 2 Cofiguration parameter (index 91).
   // ************************************************************************************************************
   36: XIO(Command_Being_Processed)XIO(Local_Control.4)EQU(LCA.Command,15)OTL(Command_Being_Processed)MOV(Port,Port_Data.Data_Transfer[185])MOV(0,Port_Data.Data_Transfer[187])MOV(91,Port_Data.Data_Transfer[188])MOV(3,Port_Data.Data_Transfer[189])OTL(Port_Data.Port_Read.[Port])OTL(Local_Control.4);
   37: XIC(Local_Control.5)XIO(Local_Control.6)EQU(LCA.Command,15)BTD(Port_Data.Data_Transfer[0],0,LCA.Write.CC_Blue,0,8)BTD(Port_Data.Data_Transfer[1],0,LCA.Write.CC2_Green,0,8)BTD(Port_Data.Data_Transfer[2],0,LCA.Write.CC2_Red,0,8)OTU(Port_Data.Port_Read.[Port])OTL(Local_Control.6);
   38: NOP();
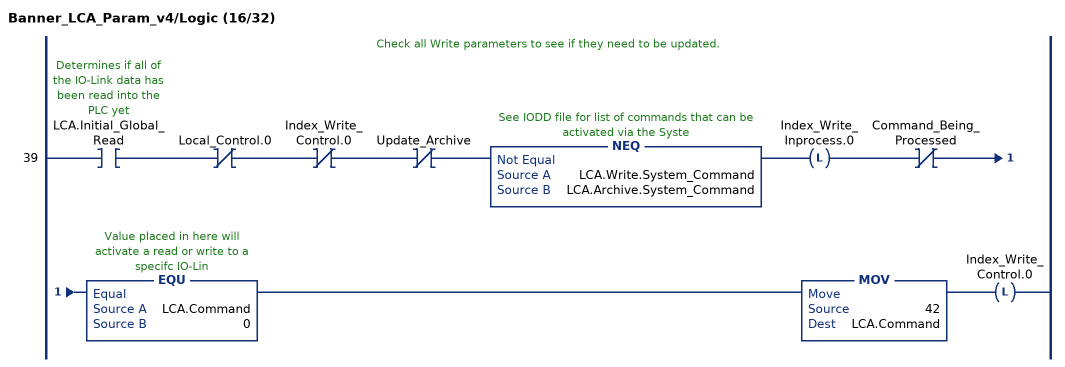
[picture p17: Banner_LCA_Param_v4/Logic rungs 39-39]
   // Check all Write parameters to see if they need to be updated.
   39: XIC(LCA.Initial_Global_Read)XIO(Local_Control.0)XIO(Index_Write_Control.0)XIO(Update_Archive)NEQ(LCA.Write.System_Command,LCA.Archive.System_Command)OTL(Index_Write_Inprocess.0)XIO(Command_Being_Processed)EQU(LCA.Command,0)MOV(42,LCA.Command)OTL(Index_Write_Control.0);
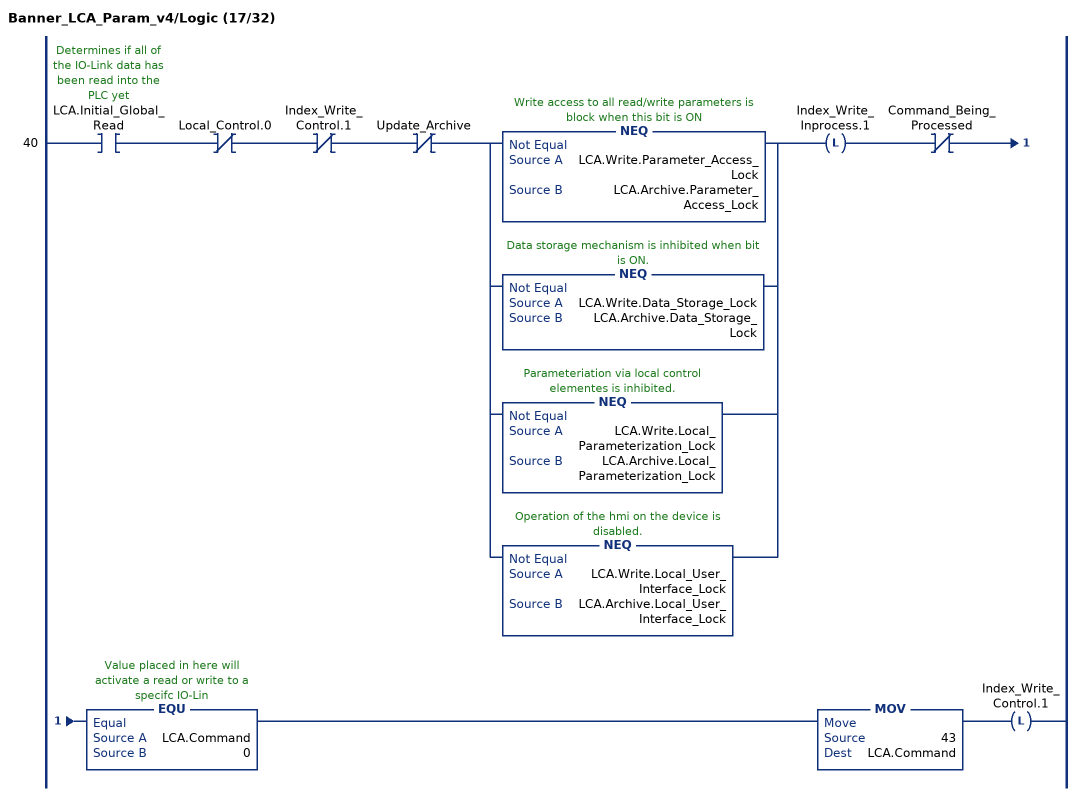
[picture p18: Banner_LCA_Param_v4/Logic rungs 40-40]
   40: XIC(LCA.Initial_Global_Read)XIO(Local_Control.0)XIO(Index_Write_Control.1)XIO(Update_Archive)[NEQ(LCA.Write.Parameter_Access_Lock,LCA.Archive.Parameter_Access_Lock) ,NEQ(LCA.Write.Data_Storage_Lock,LCA.Archive.Data_Storage_Lock) ,NEQ(LCA.Write.Local_Parameterization_Lock,LCA.Archive.Local_Parameterization_Lock) ,NEQ(LCA.Write.Local_User_Interface_Lock,LCA.Archive.Local_User_Interface_Lock) ]OTL(Index_Write_Inprocess.1)XIO(Command_Being_Processed)EQU(LCA.Command,0)MOV(43,LCA.Command)OTL(Index_Write_Control.1);
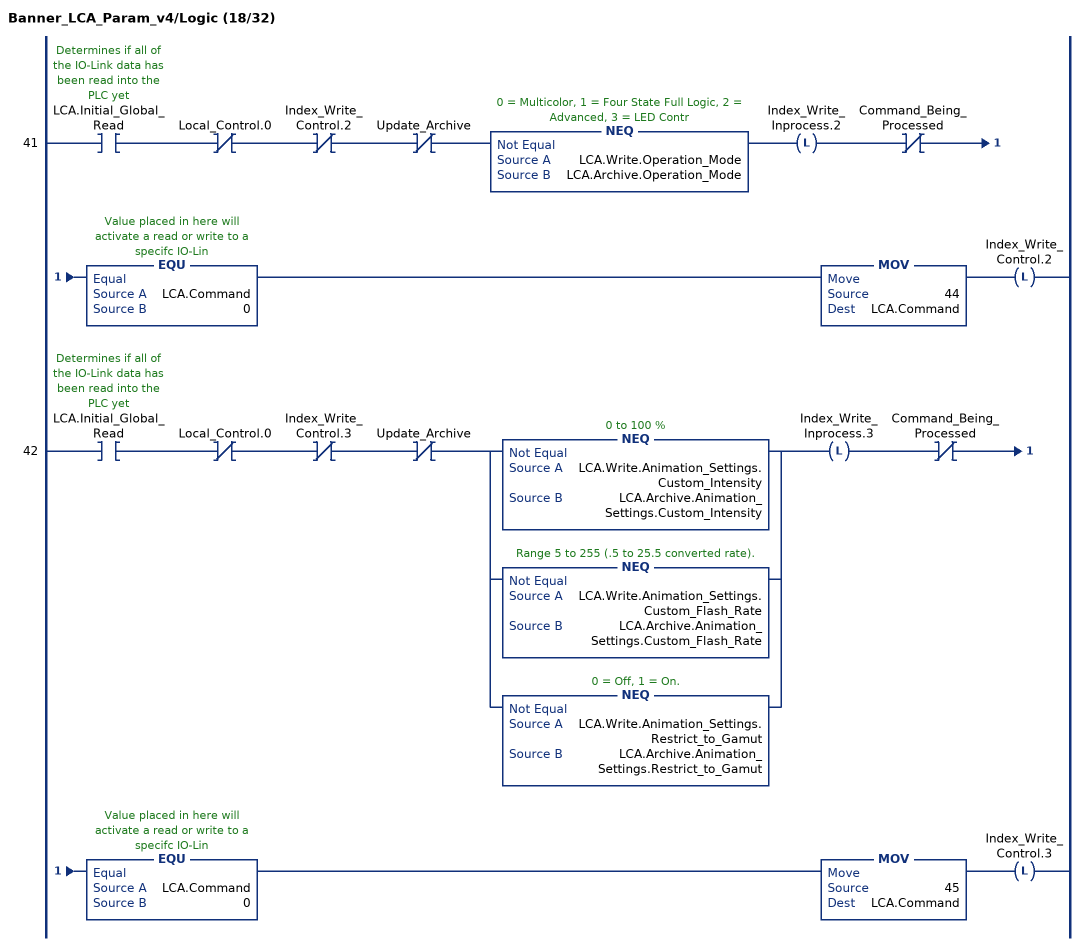
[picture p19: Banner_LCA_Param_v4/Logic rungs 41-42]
   41: XIC(LCA.Initial_Global_Read)XIO(Local_Control.0)XIO(Index_Write_Control.2)XIO(Update_Archive)NEQ(LCA.Write.Operation_Mode,LCA.Archive.Operation_Mode)OTL(Index_Write_Inprocess.2)XIO(Command_Being_Processed)EQU(LCA.Command,0)MOV(44,LCA.Command)OTL(Index_Write_Control.2);
   42: XIC(LCA.Initial_Global_Read)XIO(Local_Control.0)XIO(Index_Write_Control.3)XIO(Update_Archive)[NEQ(LCA.Write.Animation_Settings.Custom_Intensity,LCA.Archive.Animation_Settings.Custom_Intensity) ,NEQ(LCA.Write.Animation_Settings.Custom_Flash_Rate,LCA.Archive.Animation_Settings.Custom_Flash_Rate) ,NEQ(LCA.Write.Animation_Settings.Restrict_to_Gamut,LCA.Archive.Animation_Settings.Restrict_to_Gamut) ]OTL(Index_Write_Inprocess.3)XIO(Command_Being_Processed)EQU(LCA.Command,0)MOV(45,LCA.Command)OTL(Index_Write_Control.3);
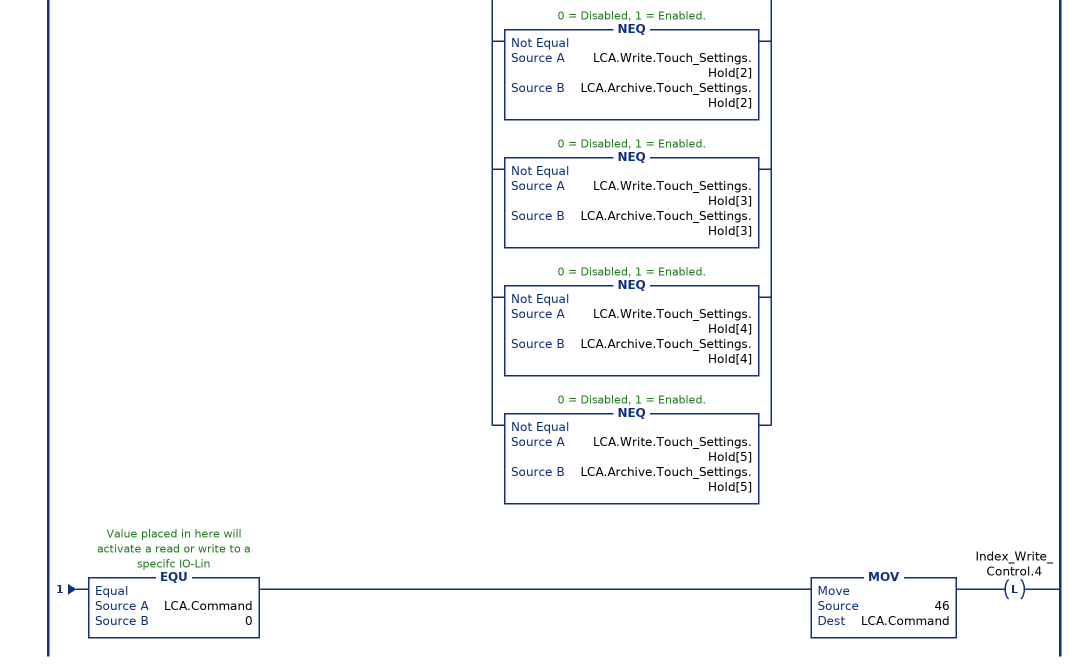
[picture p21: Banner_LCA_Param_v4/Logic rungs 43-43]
   43: XIC(LCA.Initial_Global_Read)XIO(Local_Control.0)XIO(Index_Write_Control.4)XIO(Update_Archive)[NEQ(LCA.Write.Touch_Settings.Touch_Sensitivity,LCA.Archive.Touch_Settings.Touch_Sensitivity) ,NEQ(LCA.Write.Touch_Settings.Function[1],LCA.Archive.Touch_Settings.Function[1]) ,NEQ(LCA.Write.Touch_Settings.Function[2],LCA.Archive.Touch_Settings.Function[2]) ,NEQ(LCA.Write.Touch_Settings.Function[3],LCA.Archive.Touch_Settings.Function[3]) ,NEQ(LCA.Write.Touch_Settings.Function[4],LCA.Archive.Touch_Settings.Function[4]) ,NEQ(LCA.Write.Touch_Settings.Function[5],LCA.Archive.Touch_Settings.Function[5]) ,NEQ(LCA.Write.Touch_Settings.Hold[1],LCA.Archive.Touch_Settings.Hold[1]) ,NEQ(LCA.Write.Touch_Settings.Hold[2],LCA.Archive.Touch_Settings.Hold[2]) ,NEQ(LCA.Write.Touch_Settings.Hold[3],LCA.Archive.Touch_Settings.Hold[3]) ,NEQ(LCA.Write.Touch_Settings.Hold[4],LCA.Archive.Touch_Settings.Hold[4]) ,NEQ(LCA.Write.Touch_Settings.Hold[5],LCA.Archive.Touch_Settings.Hold[5]) ]OTL(Index_Write_Inprocess.4)XIO(Command_Being_Processed)EQU(LCA.Command,0)MOV(46,LCA.Command)OTL(Index_Write_Control.4);
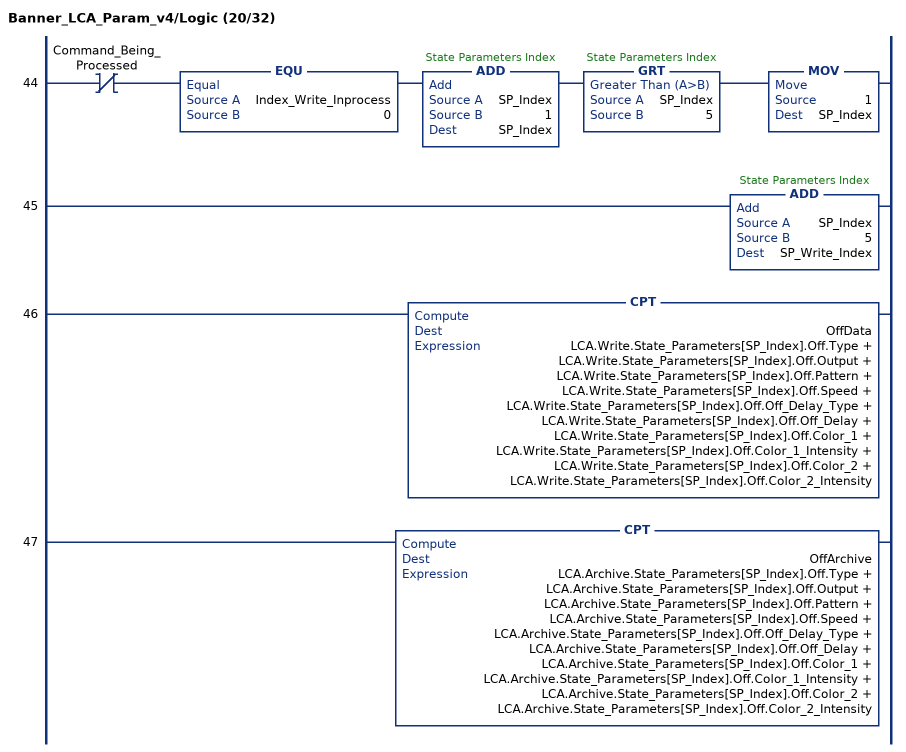
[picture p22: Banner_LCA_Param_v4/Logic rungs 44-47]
   44: XIO(Command_Being_Processed)EQU(Index_Write_Inprocess,0)ADD(SP_Index,1,SP_Index)GRT(SP_Index,5)MOV(1,SP_Index);
   45: ADD(SP_Index,5,SP_Write_Index);
   46: CPT(OffData,LCA.Write.State_Parameters[SP_Index].Off.Type + LCA.Write.State_Parameters[SP_Index].Off.Output + LCA.Write.State_Parameters[SP_Index].Off.Pattern + LCA.Write.State_Parameters[SP_Index].Off.Speed + LCA.Write.State_Parameters[SP_Index].Off.Off_Delay_Type + LCA.Write.State_Parameters[SP_Index].Off.Off_Delay + LCA.Write.State_Parameters[SP_Index].Off.Color_1 + LCA.Write.State_Parameters[SP_Index].Off.Color_1_Intensity + LCA.Write.State_Parameters[SP_Index].Off.Color_2 + LCA.Write.State_Parameters[SP_Index].Off.Color_2_Intensity);
   47: CPT(OffArchive,LCA.Archive.State_Parameters[SP_Index].Off.Type + LCA.Archive.State_Parameters[SP_Index].Off.Output + LCA.Archive.State_Parameters[SP_Index].Off.Pattern + LCA.Archive.State_Parameters[SP_Index].Off.Speed + LCA.Archive.State_Parameters[SP_Index].Off.Off_Delay_Type + LCA.Archive.State_Parameters[SP_Index].Off.Off_Delay + LCA.Archive.State_Parameters[SP_Index].Off.Color_1 + LCA.Archive.State_Parameters[SP_Index].Off.Color_1_Intensity + LCA.Archive.State_Parameters[SP_Index].Off.Color_2 + LCA.Archive.State_Parameters[SP_Index].Off.Color_2_Intensity);
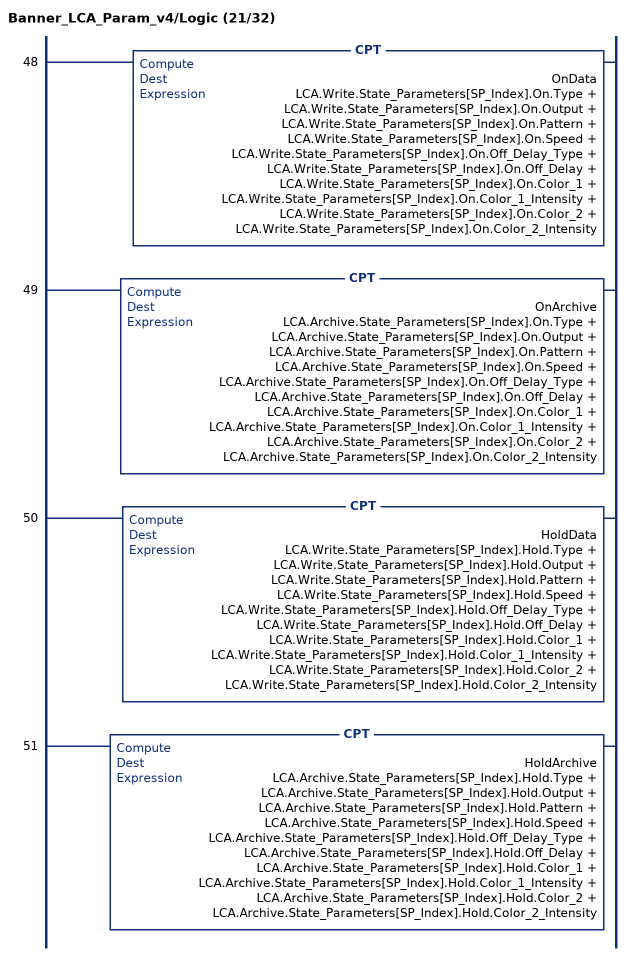
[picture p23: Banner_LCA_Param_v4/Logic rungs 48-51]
   48: CPT(OnData,LCA.Write.State_Parameters[SP_Index].On.Type + LCA.Write.State_Parameters[SP_Index].On.Output + LCA.Write.State_Parameters[SP_Index].On.Pattern + LCA.Write.State_Parameters[SP_Index].On.Speed + LCA.Write.State_Parameters[SP_Index].On.Off_Delay_Type + LCA.Write.State_Parameters[SP_Index].On.Off_Delay + LCA.Write.State_Parameters[SP_Index].On.Color_1 + LCA.Write.State_Parameters[SP_Index].On.Color_1_Intensity + LCA.Write.State_Parameters[SP_Index].On.Color_2 + LCA.Write.State_Parameters[SP_Index].On.Color_2_Intensity);
   49: CPT(OnArchive,LCA.Archive.State_Parameters[SP_Index].On.Type + LCA.Archive.State_Parameters[SP_Index].On.Output + LCA.Archive.State_Parameters[SP_Index].On.Pattern + LCA.Archive.State_Parameters[SP_Index].On.Speed + LCA.Archive.State_Parameters[SP_Index].On.Off_Delay_Type + LCA.Archive.State_Parameters[SP_Index].On.Off_Delay + LCA.Archive.State_Parameters[SP_Index].On.Color_1 + LCA.Archive.State_Parameters[SP_Index].On.Color_1_Intensity + LCA.Archive.State_Parameters[SP_Index].On.Color_2 + LCA.Archive.State_Parameters[SP_Index].On.Color_2_Intensity);
   50: CPT(HoldData,LCA.Write.State_Parameters[SP_Index].Hold.Type + LCA.Write.State_Parameters[SP_Index].Hold.Output + LCA.Write.State_Parameters[SP_Index].Hold.Pattern + LCA.Write.State_Parameters[SP_Index].Hold.Speed + LCA.Write.State_Parameters[SP_Index].Hold.Off_Delay_Type + LCA.Write.State_Parameters[SP_Index].Hold.Off_Delay + LCA.Write.State_Parameters[SP_Index].Hold.Color_1 + LCA.Write.State_Parameters[SP_Index].Hold.Color_1_Intensity + LCA.Write.State_Parameters[SP_Index].Hold.Color_2 + LCA.Write.State_Parameters[SP_Index].Hold.Color_2_Intensity);
   51: CPT(HoldArchive,LCA.Archive.State_Parameters[SP_Index].Hold.Type + LCA.Archive.State_Parameters[SP_Index].Hold.Output + LCA.Archive.State_Parameters[SP_Index].Hold.Pattern + LCA.Archive.State_Parameters[SP_Index].Hold.Speed + LCA.Archive.State_Parameters[SP_Index].Hold.Off_Delay_Type + LCA.Archive.State_Parameters[SP_Index].Hold.Off_Delay + LCA.Archive.State_Parameters[SP_Index].Hold.Color_1 + LCA.Archive.State_Parameters[SP_Index].Hold.Color_1_Intensity + LCA.Archive.State_Parameters[SP_Index].Hold.Color_2 + LCA.Archive.State_Parameters[SP_Index].Hold.Color_2_Intensity);
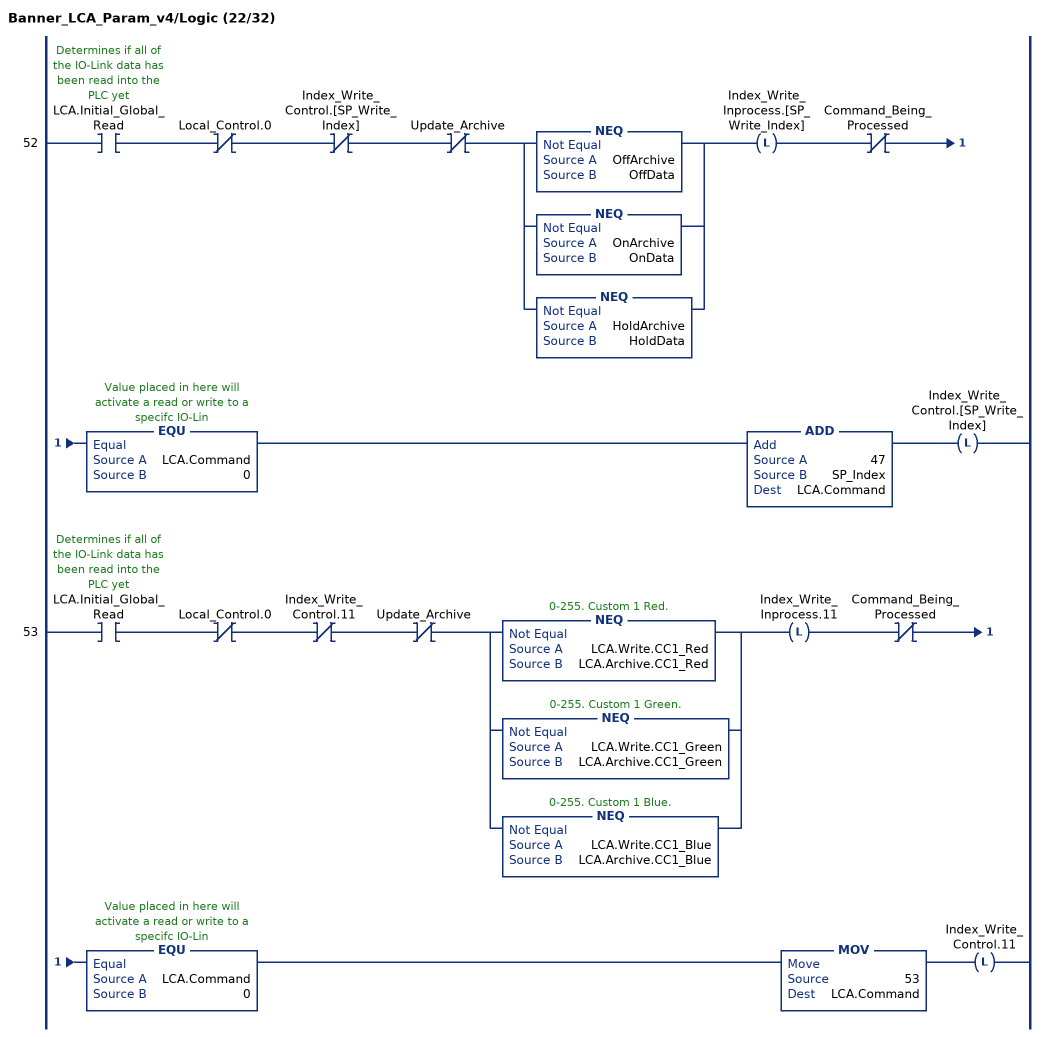
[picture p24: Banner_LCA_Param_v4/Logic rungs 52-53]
   52: XIC(LCA.Initial_Global_Read)XIO(Local_Control.0)XIO(Index_Write_Control.[SP_Write_Index])XIO(Update_Archive)[NEQ(OffArchive,OffData) ,NEQ(OnArchive,OnData) ,NEQ(HoldArchive,HoldData) ]OTL(Index_Write_Inprocess.[SP_Write_Index])XIO(Command_Being_Processed)EQU(LCA.Command,0)ADD(47,SP_Index,LCA.Command)OTL(Index_Write_Control.[SP_Write_Index]);
   53: XIC(LCA.Initial_Global_Read)XIO(Local_Control.0)XIO(Index_Write_Control.11)XIO(Update_Archive)[NEQ(LCA.Write.CC1_Red,LCA.Archive.CC1_Red) ,NEQ(LCA.Write.CC1_Green,LCA.Archive.CC1_Green) ,NEQ(LCA.Write.CC1_Blue,LCA.Archive.CC1_Blue) ]OTL(Index_Write_Inprocess.11)XIO(Command_Being_Processed)EQU(LCA.Command,0)MOV(53,LCA.Command)OTL(Index_Write_Control.11);
